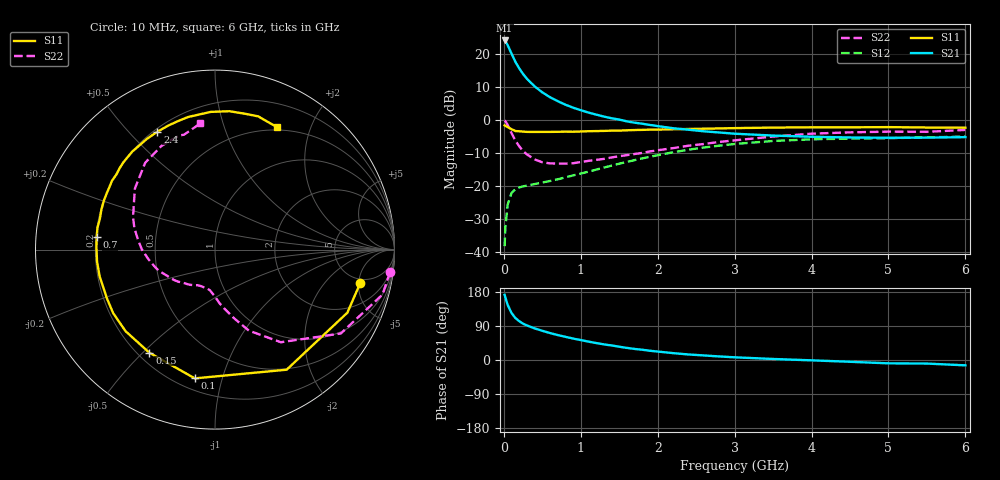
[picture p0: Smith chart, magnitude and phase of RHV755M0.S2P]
! SIEMENS Small Signal Semiconductors
! BFR106
! Si NPN RF Bipolar Junction Transistor in SOT23
! VCE = 0.75 V  IC = 5 mA
! Common Emitter S-Parameters:  August  1996
# GHz  S  MA  R  50
!  f  S11  S21  S12  S22
! GHz  MAG  ANG  MAG  ANG  MAG  ANG  MAG  ANG
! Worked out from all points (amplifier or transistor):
!   36 points, 10 MHz to 6 GHz, reference 50 ohm
!   highest |S21| = 24.1 dB at 10 MHz (marker M1)
!   |S21| within 3 dB of that: start of sweep to 80.49 MHz
!   unconditionally stable (mu >= 1): 580.2 MHz to end of sweep
!   at 250 MHz: K = 0.52, MSG = 17.0 dB, |S12| = -20.1 dB
!   at 1.4 GHz: K = 1.20, MAG = 4.5 dB, |S12| = -13.8 dB
!   at 6 GHz: K = 1.03, MAG = -1.1 dB, |S12| = -5.0 dB
!   S11 on the Smith chart (normalised r, x): 10 MHz: 4.35, -5.24; 100 MHz: 0.27, -0.82; 150 MHz: 0.24, -0.52; 700 MHz: 0.20, +0.05; 2.4 GHz: 0.21, +0.60; 6 GHz: 0.46, +1.52
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0.01  0.8304 -13.0  16.11 171.8  0.0122 83.6  0.9831 -7.4
0.02  0.8169 -25.5  15.72 165.0  0.0239 77.4  0.9665 -15.0
0.05  0.7791 -59.2  13.63 145.2  0.0523 60.4  0.8424 -33.7
0.1  0.7262 -98.9  10.18 124.1  0.0783 44.3  0.6331 -54.6
0.15  0.681 -122.5  7.646 110.7  0.089 36.0  0.4894 -67.3
0.2  0.6744 -137.6  6.085 102.4  0.0947 32.5  0.3999 -74.2
0.25  0.6688 -148.1  4.985 95.8  0.0985 30.7  0.3372 -80.4
0.3  0.6606 -155.8  4.221 91.2  0.1014 30.8  0.3012 -85.0
0.4  0.6598 -166.8  3.239 83.5  0.1068 31.8  0.2527 -91.7
0.5  0.6606 -174.2  2.626 77.0  0.1128 33.8  0.2287 -97.0
0.6  0.6606 179.1  2.221 71.1  0.1189 36.5  0.22 -102.2
0.7  0.6629 173.9  1.934 65.8  0.126 39.1  0.2186 -107.6
0.9  0.6638 165.1  1.54 56.6  0.1444 43.4  0.221 -116.3
1.1  0.6765 156.4  1.298 48.5  0.1649 46.6  0.2402 -125.3
1.3  0.6839 149.2  1.128 41.2  0.1899 48.6  0.2569 -134.3
1.6  0.6985 139.6  0.954 31.9  0.2318 49.1  0.2937 -147.1
2.2  0.7242 121.7  0.751 18.1  0.324 43.9  0.3748 -171.7
2.4  0.7312 116.0  0.713 14.6  0.3547 41.0  0.4078 179.8
3.5  0.7677 91.7  0.581 2.7  0.481 22.0  0.5612 142.7
4.5  0.7751 77.6  0.544 -4.7  0.5229 6.1  0.6501 117.3
5.5  0.7696 67.4  0.541 -9.4  0.5461 -3.2  0.6628 105.1
6  0.7655 63.4  0.55 -14.1  0.561 -9.8  0.7074 96.7
